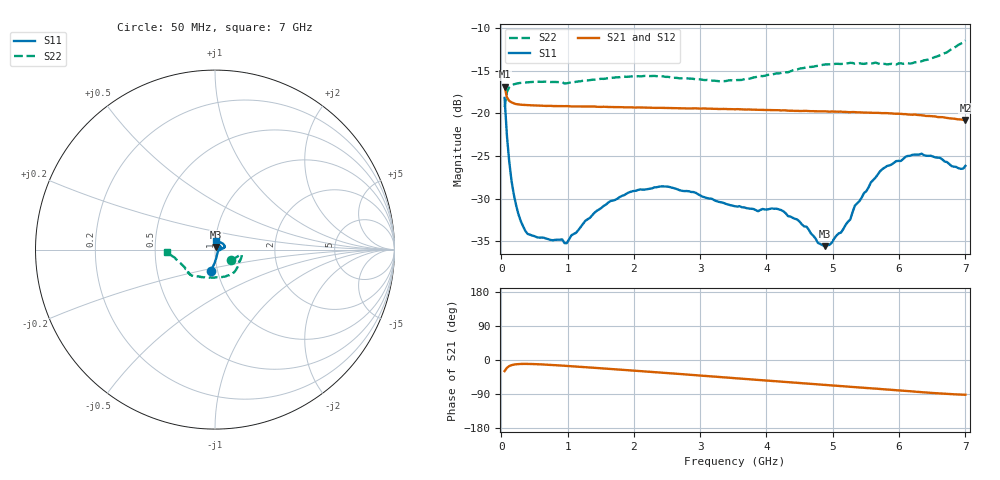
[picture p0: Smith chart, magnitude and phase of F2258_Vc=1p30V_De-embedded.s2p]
! Integrated Device Technology
! Corporate Headquarters
! 6024 Silver Creek Valley Road
! San Jose, CA 95138  USA
! Phone:  1-408-284-8200
! Toll Free:  1-800-223-1366
! Webpage:  http://www.idt.com/
! Timing and RF Division
! 515 Groton Road, Suite 102
! Westford, MA 01886-6024
! Device:  F2258
! Description: Voltage Variable RF Attenuator
! Frequency:  50.0 -  6000.00 MHz
! Package:  3x3 mm Thin QFN Plastic Package: 16 pin
! Ports:  2 RF, 2 DC
!  Pin  1  = NC
!  Pin  2  = NC
!  Pin  3  = RF2  = Port 2
!  Pin  4  = GND
!  Pin  5  = Vdd
!  Pin  6  = NC
!  Pin  7  = VCTRL
!  Pin  8  = NC
!  Pin  9  = GND
!  Pin 10  = RF1  = Port 1
!  Pin 11  = NC
!  Pin 12  = NC
!  Pin 13  = NC
!  Pin 14  = NC
!  Pin 15  = NC
!  Pin 16  = NC
! Vcntrl:  1.300 Volts
! Vdd:  +3.300 Volts
! Current:  1.167 mA
! Data:  The device was measured on a the F2258 evaluation board which has
!  individual transmission lines to the RF pins.  Data was collected
!  using a calibrated network analyzer.  The evaluation board was
!  de-embedded using a TRL calibration technique.
!  The reference plane is the edge of the package pin.
! Misc:  SN 10
!  Action Tracker AT0285
! Date Measured:  2014-12-10
! Date:  2016-01-13  MJV
! Note:
!  Integrated Device Technology supplies this data as a sample of measured
!  data at the package pin for this product.  Your particular data for this
!  product may vary.
!  Data was taken at 25 degrees C.
!  Integrated Device Technology reserves the right to change this data at anytime.
!Freq_(GHz)  S11M_(dB)  S11P_(deg)  S21M_(dB)  S21P_(deg)  S12M_(dB)  S12P_(deg)  S22M_(dB)  S22P_(deg)
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# GHz S dB R 50
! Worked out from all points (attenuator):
!   201 points, 50 MHz to 7 GHz, reference 50 ohm
!   highest |S21| = -16.87 dB at 50 MHz (marker M1); lowest = -20.8 dB at 7 GHz (marker M2)
!   lowest |S11| = -35.6 dB at 4.88 GHz (marker M3), VSWR 1.03, Z = 50.7 + j1.51 ohm
!   |S11| at or under -10 dB: start of sweep to end of sweep
!   |S22| runs from -19.3 to -11.5 dB; largest |S21 - S12| = 0.00041
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0.05  -18.19 -101.1  -16.87 -29.2  -16.85 -29.2  -19.28 -33.2
0.08475  -22.59 -91.5  -18.13 -20.5  -18.10 -20.5  -17.51 -16.0
0.15425  -27.90 -78.0  -18.71 -13.6  -18.74 -13.6  -16.72 -10.9
0.2585  -31.81 -61.4  -18.95 -10.7  -18.95 -10.7  -16.47 -10.5
0.36275  -33.77 -47.7  -19.03 -10.3  -19.02 -10.3  -16.38 -12.1
0.98825  -35.20 -20.9  -19.15 -15.6  -19.16 -15.6  -16.48 -26.9
1.2315  -32.96 -10.4  -19.19 -18.4  -19.18 -18.4  -16.18 -32.4
1.6485  -30.27 -1.9  -19.25 -23.7  -19.25 -23.7  -15.85 -41.6
2.37825  -28.59 15.8  -19.35 -32.9  -19.37 -32.9  -15.64 -57.5
3.525  -30.88 68.5  -19.52 -48.0  -19.52 -48.0  -16.13 -94.9
4.22  -31.32 97.8  -19.66 -57.1  -19.65 -57.2  -15.26 -118.6
4.60225  -33.26 93.0  -19.71 -62.1  -19.74 -62.0  -14.58 -126.8
4.7065  -34.34 83.0  -19.74 -63.4  -19.74 -63.4  -14.53 -128.3
4.88025  -35.55 63.2  -19.76 -65.8  -19.77 -65.7  -14.28 -130.6
5.1235  -33.96 33.5  -19.79 -68.9  -19.82 -68.8  -14.22 -133.5
5.2625  -32.44 19.8  -19.86 -70.6  -19.87 -70.6  -14.08 -135.1
5.332  -30.82 16.0  -19.85 -71.6  -19.87 -71.6  -14.17 -135.4
5.57525  -28.08 10.0  -19.92 -74.7  -19.91 -74.7  -14.18 -139.0
5.85325  -26.10 10.7  -20.00 -78.4  -19.99 -78.4  -14.23 -143.5
6.33975  -24.72 20.9  -20.23 -85.0  -20.22 -85.0  -13.90 -155.6
6.89575  -26.43 68.9  -20.70 -91.1  -20.72 -91.0  -11.97 -173.9
7  -26.15 84.1  -20.78 -91.7  -20.76 -91.7  -11.46 -177.2
